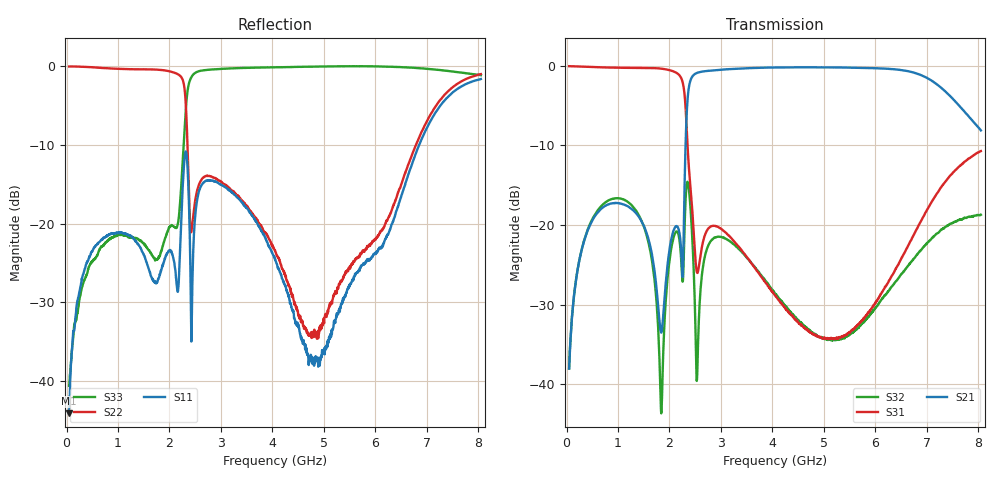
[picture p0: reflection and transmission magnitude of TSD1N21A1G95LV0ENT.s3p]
# MHZ S RI R 50
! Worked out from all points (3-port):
!   1601 points, 50 MHz to 8.05 GHz, reference 50 ohm
!   strongest paths, dB at 50 MHz, 2.05 GHz, 4.05 GHz, 6.05 GHz, 8.05 GHz:
!     S21: -38.0, -21.3, -0.2, -0.3, -8.1
!     S31: 0.0, -0.6, -28.8, -29.3, -10.7
!     S32: -38.0, -22.4, -28.6, -30.0, -18.7
!   lowest |S11| = -44.1 dB at 50 MHz (marker M1), VSWR 1.01, Z = 49.9 - j0.608 ohm
!   |S11| at or under -10 dB: start of sweep to 6.852 GHz
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50  -0.00124 -0.00609  0.000833 0.0125  0.9904 -0.0492
    0.000909 0.0125  0.9897 -0.1143  0.00128 0.0126
    0.9946 -0.0493  0.00124 0.0125  0.00749 -0.0055
730  -0.0646 -0.0495  0.1015 0.0827  0.7495 -0.6287
     0.1013 0.0827  0.0134 -0.9733  0.1353 0.0196
     0.7493 -0.6289  0.1356 0.0193  -0.0212 -0.0711
1540  -0.0106 0.0577  0.0913 0.0137  -0.0722 -0.9661
      0.091 0.0139  -0.9469 -0.1256  0.00495 -0.0892
      -0.0738 -0.9681  0.00463 -0.0897  -0.00522 -0.0722
1840  0.0453 -0.0231  0.00906 0.0192  -0.5472 -0.7879
      0.00884 0.0192  -0.8116 0.4881  -0.00495 0.00426
      -0.548 -0.7891  -0.00498 0.00429  0.0474 -0.0474
2285  0.2239 -0.0937  -0.0921 -0.0913  -0.4437 0.5384
      -0.0923 -0.0916  0.6409 0.3867  0.0779 0.00677
      -0.4429 0.5377  0.0776 0.00668  0.2414 0.2611
2630  0.028 -0.1746  0.0704 0.915  -0.0697 -0.0227
      0.07 0.9165  0.0674 0.18  0.049 0.0044
      -0.0694 -0.0224  0.0486 0.00418  0.6563 -0.6713
4050  -0.0583 0.00969  0.9528 -0.2087  -0.036 0.00485
      0.9549 -0.2102  0.0658 -0.0157  -0.0228 -0.0299
      -0.0359 0.00468  -0.0226 -0.0296  -0.5482 -0.8179
4900  -0.0106 0.00777  0.6688 -0.7148  -0.0174 0.00931
      0.6683 -0.7149  0.00971 -0.0187  -0.0189 -0.00617
      -0.0174 0.00935  -0.0188 -0.00644  -0.8158 -0.5695
6055  0.0642 0.0228  -0.082 -0.9614  -0.0268 0.0211
      -0.0808 -0.9618  0.0658 -0.0507  -0.0226 0.0219
      -0.027 0.0214  -0.0227 0.0225  -0.9386 -0.3374
8050  -0.783 0.2743  -0.3688 0.1361  0.1558 0.252
      -0.3681 0.1389  0.7474 -0.4864  0.116 -0.0205
      0.1543 0.2478  0.1143 -0.0195  -0.5428 0.6889
